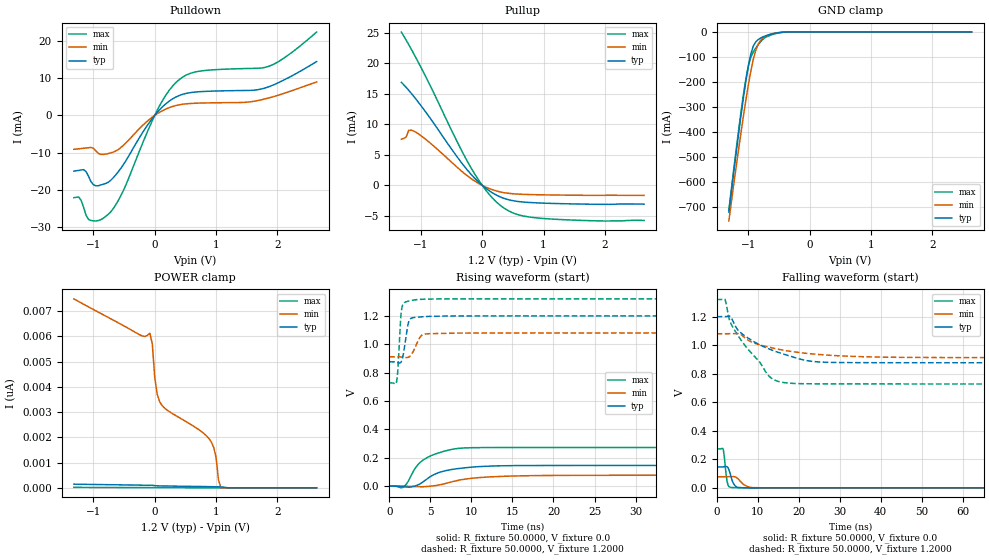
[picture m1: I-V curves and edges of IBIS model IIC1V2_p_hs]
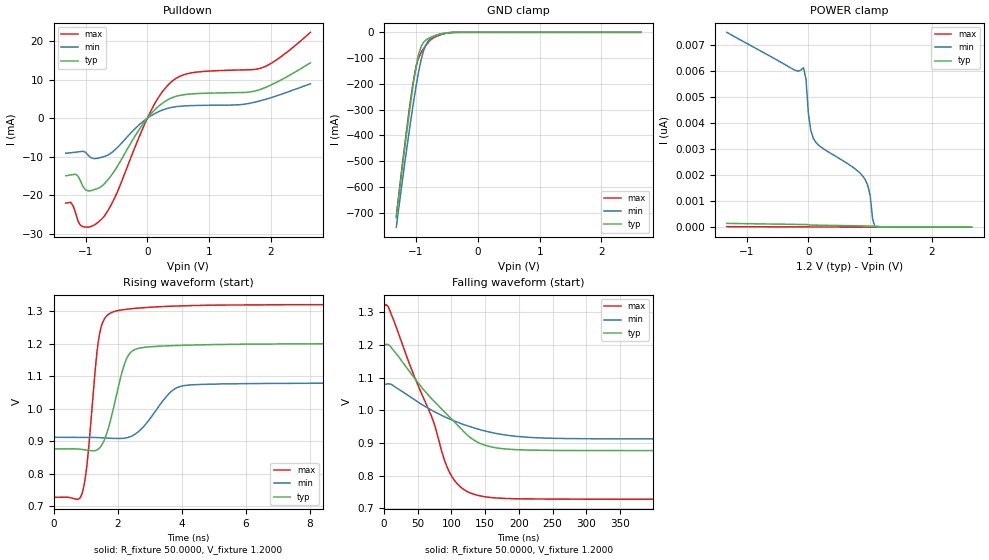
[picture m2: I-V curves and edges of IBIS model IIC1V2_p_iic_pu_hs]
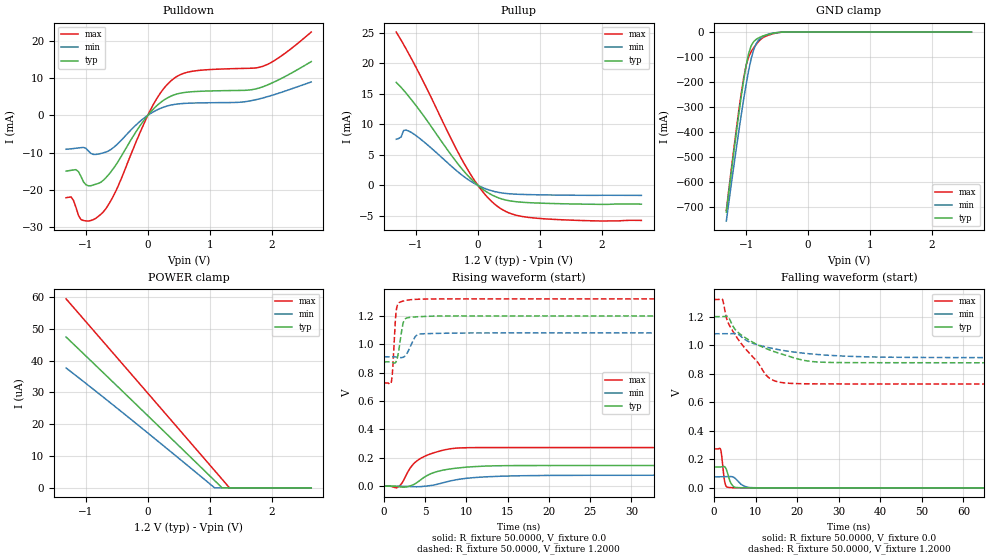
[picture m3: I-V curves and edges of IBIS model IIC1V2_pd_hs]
| IBIS file qfp64afe_1p2v.ibs generated by Viper version: 2020.12.17
[IBIS Ver]   5.0
[Comment Char]   |_char
[File Name]   qfp64afe_1p2v.ibs
[File Rev]   1.3
[Date]   Thu Dec 17 17:47:12 2020
[Source]   NXP Viper 2020.12.17
[Notes]
[Disclaimer] IMPORTANT NOTICE
  This information is provided on an AS IS basis and without warranty.
  IN NO EVENT SHALL NXP BE LIABLE FOR INCIDENTAL OR CONSEQUENTIAL
  DAMAGES ARISING FROM USE OF THIS INFORMATION. THIS DISCLAIMER OF
  WARRANTY EXTENDS TO THE USER OF THE INFORMATION, AND TO THEIR CUSTOMERS
  OR USERS OF PRODUCTS  AND IS IN LIEU OF ALL WARRANTIES WHETHER EXPRESS,
  IMPLIED, OR STATUTORY, INCLUDING IMPLIED WARRANTIES OF MERCHANTABILITY
  OR FITNESS FOR PARTICULAR PURPOSE.
  NXP does not represent or warrant that the information furnished
  hereunder is free of infringement of any third party patents,
  copyrights, trade secrets, or other intellectual property rights.
  NXP does not represent or warrant that the information is free of
  defect, or that it meets any particular standard, requirements or need
  of the user of the infomation or their customers.
  NXP reserves the right to change the information in this file
  without notice.
   http://www.nxp.com
[Copyright]   (C) Copyright NXP 2004 - 2020, All Rights Reserved.
|   qfp64Afe
[Component]   qfp64Afe
[Manufacturer]   NXP
[Package]
| variable   typ   min   max
R_pkg   0.18002   0.098036   0.22836
L_pkg   3.270e-09   2.478e-09   3.882e-09
C_pkg   4.877e-13   4.194e-13   6.388e-13
[Pin] signal_name   model_name   R_pin   L_pin   C_pin
1   P2_1   gpio   0.20176   3.768e-09 4.934e-13
2   OPAMP2_INN   NC   0.18655   3.432e-09 5.614e-13
3   P0_1   gpio   0.1882   3.425e-09 5.543e-13
4   P1_0   gpio   0.18167   3.391e-09 4.852e-13
5   ADC1IN1B   NC   0.17508   3.272e-09 4.734e-13
6   ADC1IN1A   NC   0.17211   3.184e-09 4.709e-13
7   P0_11   gpio   0.17322   3.095e-09 4.516e-13
8   VDDA   POWER   NA   NA   NA
9   VREF_OUT   NC   0.098933  2.478e-09 5.107e-13
10   VREFP   NC   0.098036  2.682e-09 4.989e-13
11   VREFN   NC   0.10339   2.593e-09 5.200e-13
12   VSSA   GND   NA   NA   NA
13   P0_16   gpio   0.18219   3.272e-09 4.683e-13
14   P0_10   gpio   0.18473   3.372e-09 4.943e-13
15   P0_15   gpio   0.1948   3.518e-09 5.647e-13
16   P0_31   gpio   0.21166   3.882e-09 5.047e-13
17   P0_8   gpio   0.19981   3.690e-09 4.818e-13
18   OPAMP0_INN   NC   0.18485   3.354e-09 5.404e-13
19   P0_27   gpio   0.1771   3.251e-09 5.158e-13
20   OPAMP1_INN   NC   0.17264   3.242e-09 4.518e-13
21   XTAL32M_N   NC   0.17308   3.207e-09 4.514e-13
22   XTAL32M_P   NC   0.17099   3.143e-09 4.435e-13
23   RESETN   gpio   0.17312   3.058e-09 4.290e-13
24   VDD_CORE   POWER   NA   NA   NA
25   P1_22   gpio   0.17347   2.976e-09 4.359e-13
26   P0_17   gpio   0.17222   3.063e-09 4.368e-13
27   P0_7   gpio   0.17974   2.960e-09 4.541e-13
28   VDDE_2   POWER   NA   NA   NA
29   VSS_MAIN_PWR   GND   NA   NA   NA
30   VSS_MAIN   GND   NA   NA   NA
31   LX   NC   0.12471   2.527e-09 6.388e-13
32   VDD_MAIN_PWR   NC   NA   NA   NA
33   XTAL32K_P   NC   0.20305   3.722e-09 4.831e-13
34   XTAL32K_N   NC   0.18797   3.388e-09 5.425e-13
35   VBAT   NC   0.17937   3.272e-09 4.763e-13
36   P0_0   gpio   0.17575   3.216e-09 4.542e-13
37   P0_9   gpio   0.17142   3.151e-09 4.522e-13
38   P0_18   gpio   0.17027   3.108e-09 4.408e-13
39   P1_13   gpio   0.17092   3.083e-09 4.194e-13
40   P1_1   gpio   0.17351   3.079e-09 4.367e-13
41   P0_26   gpio   0.17937   3.140e-09 4.480e-13
42   P1_2   gpio   0.18924   3.260e-09 4.417e-13
43   P1_3   gpio   0.20575   3.278e-09 4.623e-13
44   VDDE_4   POWER   NA   NA   NA
45   P0_24   gpio   0.18768   3.277e-09 4.591e-13
46   P0_13   iic   0.19613   3.445e-09 5.506e-13
47   P0_14   iic   0.20782   3.616e-09 5.657e-13
48   P0_20   gpio   0.21594   3.876e-09 4.850e-13
49   P0_21   gpio   0.20723   3.837e-09 4.904e-13
50   P0_22   gpio   0.1962   3.547e-09 5.661e-13
51   P0_25   gpio   0.18792   3.420e-09 5.062e-13
52   P0_2   gpio   0.18663   3.397e-09 4.750e-13
53   P1_15   gpio   0.17882   3.273e-09 4.700e-13
54   P0_19   gpio   0.17446   3.156e-09 4.633e-13
55   P0_3   gpio   0.17673   3.008e-09 4.457e-13
56   VDDE_4   POWER   NA   NA   NA
57   P0_4   gpio   0.17637   3.003e-09 4.457e-13
58   P1_16   gpio   0.17537   3.170e-09 4.476e-13
59   P0_6   gpio   0.17935   3.248e-09 4.687e-13
60   P0_5   gpio   0.18758   3.378e-09 4.757e-13
61   P0_29   gpio   0.19171   3.430e-09 4.834e-13
62   P1_11   gpio   0.20582   3.539e-09 5.647e-13
63   P0_30   gpio   0.22836   3.428e-09 5.818e-13
64   VDDE_4   POWER   NA   NA   NA
65   VSS   GND   NA   NA   NA
[Pin Mapping]   pulldown_ref   pullup_ref
1   VSS   VDDA
2   NC   NC
3   VSS   VDDA
4   VSS   VDDA
5   NC   NC
6   NC   NC
7   VSS   VDDA
8   NC   VDDA
9   NC   NC
10   NC   NC
11   NC   NC
12   VSSA   NC
13   VSS   VDDA
14   VSS   VDDA
15   VSS   VDDA
16   VSS   VDDA
17   VSS   VDDA
18   NC   NC
19   VSS   VDDA
20   NC   NC
21   NC   NC
22   NC   NC
23   VSS   VDDE_2
24   NC   VDD_CORE
25   VSS   VDDE_2
26   VSS   VDDE_2
27   VSS   VDDE_2
28   NC   VDDE_2
29   VSS_MAIN_PWR   NC
30   VSS_MAIN   NC
31   NC   NC
32   NC   NC
33   NC   NC
34   NC   NC
35   NC   NC
36   VSS   VDDE_4
37   VSS   VDDE_4
38   VSS   VDDE_4
39   VSS   VDDE_4
40   VSS   VDDE_4
41   VSS   VDDE_4
42   VSS   VDDE_4
43   VSS   VDDE_4
44   NC   VDDE_4
45   VSS   VDDE_4
46   VSS   VDDE_4
47   VSS   VDDE_4
48   VSS   VDDE_4
49   VSS   VDDE_4
50   VSS   VDDE_4
51   VSS   VDDE_4
52   VSS   VDDE_4
53   VSS   VDDE_4
54   VSS   VDDE_4
55   VSS   VDDE_4
56   NC   VDDE_4
57   VSS   VDDE_4
58   VSS   VDDE_4
59   VSS   VDDE_4
60   VSS   VDDE_4
61   VSS   VDDE_4
62   VSS   VDDE_4
63   VSS   VDDE_4
64   NC   VDDE_4
65   VSS   NC
|*   Model Selector   *
[Model Selector] gpio
MFIO1V2_pd_hs   EPUN=1 EPD=1 EHS=1
MFIO1V2_pd_ls   EPUN=1 EPD=1 EHS=0
MFIO1V2_pu_hs   EPUN=0 EPD=0 EHS=1
MFIO1V2_pu_ls   EPUN=0 EPD=0 EHS=0
MFIO1V2_p_hs   EPUN=1 EPD=0 EHS=1
MFIO1V2_p_ls   EPUN=1 EPD=0 EHS=0
MFIO1V2_r_hs   EPUN=0 EPD=1 EHS=1
MFIO1V2_r_ls   EPUN=0 EPD=1 EHS=0
[Model Selector] iic
IIC1V2_pd_hs   EGP=1 EPUN=1 EPD=1 EHS=1
IIC1V2_pd_ls   EGP=1 EPUN=1 EPD=1 EHS=0
IIC1V2_p_hs   EGP=1 EPUN=1 EPD=0 EHS=1
IIC1V2_p_ls   EGP=1 EPUN=1 EPD=0 EHS=0
IIC1V2_pu_hs   EGP=1 EPUN=0 EPD=0 EHS=1
IIC1V2_pu_ls   EGP=1 EPUN=0 EPD=0 EHS=0
IIC1V2_r_hs   EGP=1 EPUN=0 EPD=1 EHS=1
IIC1V2_r_ls   EGP=1 EPUN=0 EPD=1 EHS=0
IIC1V2_pd_iic_hs   EGP=0 ECS=0 EPUN=1 EPD=1
IIC1V2_p_iic_hs   EGP=0 ECS=0 EPUN=1 EPD=0
IIC1V2_pu_iic_hs   EGP=0 ECS=0 EPUN=0 EPD=0
IIC1V2_r_iic_hs   EGP=0 ECS=0 EPUN=0 EPD=1
IIC1V2_pd_iic_pu_hs   EGP=0 ECS=1 EPUN=1 EPD=1 SSEL=1
IIC1V2_p_iic_pu_hs   EGP=0 ECS=1 EPUN=1 EPD=0 SSEL=1
IIC1V2_pu_iic_pu_hs   EGP=0 ECS=1 EPUN=0 EPD=0 SSEL=1
IIC1V2_r_iic_pu_hs   EGP=0 ECS=1 EPUN=0 EPD=1 SSEL=1
| End [Component] qfp64Afe
| Models and submodels in the file (24): IIC1V2_p_hs (I/O), IIC1V2_p_iic_hs (I/O_open_drain), IIC1V2_p_iic_pu_hs (I/O_open_drain), IIC1V2_p_ls (I/O), IIC1V2_pd_hs (I/O), IIC1V2_pd_iic_hs (I/O_open_drain), IIC1V2_pd_iic_pu_hs (I/O_open_drain), IIC1V2_pd_ls (I/O), IIC1V2_pu_hs (I/O), IIC1V2_pu_iic_hs (I/O_open_drain), IIC1V2_pu_iic_pu_hs (I/O_open_drain), IIC1V2_pu_ls (I/O), IIC1V2_r_hs (I/O), IIC1V2_r_iic_hs (I/O_open_drain), IIC1V2_r_iic_pu_hs (I/O_open_drain), IIC1V2_r_ls (I/O), MFIO1V2_p_hs (I/O), MFIO1V2_p_ls (I/O), MFIO1V2_pd_hs (I/O), MFIO1V2_pd_ls (I/O), MFIO1V2_pu_hs (I/O), MFIO1V2_pu_ls (I/O), MFIO1V2_r_hs (I/O), MFIO1V2_r_ls (I/O)
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[Model] IIC1V2_p_hs
|   Model IIC1V2_p_hs
| This model was characterised for following simulation conditions:
| External (pad) voltage:
|   - Typ: 1.2V,   - Min: 1.08V,   - Max: 1.32V
| Library cells for typ/min/max conditions are connected as defined below:
|  IO - External Pad
|  A - Core Input
|  EN - Output Buffer Enable
|  BOOST - vdde
|  EGP - vdd
|  EHS - vdd
|  ENZI - vdd
|  EPD - gnd
|  EPUN - vdd
|  ZI - NC
|  ZIF - NC
|  gnd - gnd
|  gnde - gnde
|  vdd - vdd
|  vdde - vdde
| All other pins connected to ground
Model_type I/O
Polarity   Non-Inverting
Enable   Active-Low
Vinl =   0.5400V
Vinh =   1.2600V
Vmeas =  0.9000V
Cref =   0.0F
Rref =   1.0000k
Vref =   0.0V
C_comp   3.6473pF   3.5138pF   3.7665pF
|C_comp_pullup   0.9539pF   0.9082pF   0.9728pF
|C_comp_pulldown   2.3399pF   2.4915pF   2.1962pF
[Model Spec]
| variable   typ   min   max
Vinh   0.3600V   0.3240V   0.3960V
Vinl   0.8400V   0.7560V   0.9240V
Vmeas   0.6000V   0.5400V   0.6600V
[Temperature Range]   25.0000   0.1250k   -40.0000
[Voltage Range]   1.2000V   1.0800V   1.3200V
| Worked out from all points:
|   slope of the pulldown table from 0 to 0.18 V, typ, clamps not added: 58.3 ohm
|   slope of the pullup table from 0 to 0.18 V, typ, clamps not added: 138 ohm
|   GND clamp passes 1 mA (typ) near -0.45 V on its own axis
|   rising waveform, R_fixture 50.0000, V_fixture 0.0: 20-80 % time 3.45ns typ, 4.61ns min, 2.73ns max; typ from 0 V to 0.146 V
|   rising waveform, R_fixture 50.0000, V_fixture 1.2000: 20-80 % time 519ps typ, 830ps min, 343ps max; typ from 0.877 V to 1.2 V
|   falling waveform, R_fixture 50.0000, V_fixture 0.0: 20-80 % time 1.02ns typ, 1.79ns min, 624ps max; typ from 0.146 V to 0 V
|   falling waveform, R_fixture 50.0000, V_fixture 1.2000: 20-80 % time 11.4ns typ, 13.9ns min, 8.37ns max; typ from 1.2 V to 0.877 V
[Pulldown]
|Voltage   I(typ)   I(min)   I(max)
-1.32V    -14.96mA   -9.099mA   -22.09mA
-1.24V    -14.75mA   -8.982mA   -21.89mA
-1.16V    -14.56mA   -8.83mA    -24.7mA
-1.04V    -17.82mA   -8.609mA   -28.21mA
-920mV    -18.88mA   -10.21mA   -28.21mA
-720mV    -17.44mA   -10.07mA   -25.94mA
-520mV    -13.41mA   -8.157mA   -20.44mA
80mV      1.521mA    840uA      2.628mA
440mV     5.569mA    2.951mA    10.1mA
760mV     6.377mA    3.307mA    11.92mA
1.84V     7.559mA    4.586mA    13.06mA
2.64V     14.43mA    8.958mA    22.36mA
[Pullup]
|Voltage   I(typ)   I(min)   I(max)
-1.32V    16.87mA    7.562mA    25.11mA
-1.24V    16.04mA    7.944mA    23.76mA
-1.2V     15.58mA    9.001mA    23.05mA
-1.08V    14.1mA     8.693mA    20.85mA
-400mV    4.54mA     2.884mA    6.955mA
-200mV    2.009mA    1.241mA    3.176mA
80mV      -640.3uA   -373.7uA   -1.07mA
320mV     -1.996mA   -1.123mA   -3.467mA
560mV     -2.602mA   -1.412mA   -4.719mA
920mV     -2.876mA   -1.532mA   -5.352mA
1.96V     -3.103mA   -1.628mA   -5.823mA
2.64V     -3.069mA   -1.636mA   -5.736mA
[GND_clamp]
|Voltage   I(typ)   I(min)   I(max)
-1.32V    -720.7mA   -756.4mA   -713.8mA
-1.12V    -330.9mA   -399.5mA   -316.8mA
-1.04V    -192.4mA   -269.2mA   -184.4mA
-1V       -133.6mA   -209.3mA   -133.5mA
-960mV    -86.73mA   -154.7mA   -99.45mA
-920mV    -55.68mA   -108.2mA   -79.01mA
-880mV    -39.01mA   -72.34mA   -63.7mA
-840mV    -29.9mA    -47.99mA   -50.25mA
-760mV    -18.92mA   -23.38mA   -28.31mA
-640mV    -9.212mA   -8.622mA   -12.72mA
-400mV    -328.4uA   -396.6uA   -434.3uA
2.64V     0A         0A         0A
[POWER_clamp]
|Voltage   I(typ)   I(min)   I(max)
-1.32V    146.2pA    7.487nA    20.6pA
-240mV    107.2pA    6.058nA    10.71pA
-80mV     104.3pA    6.128nA    10.43pA
-40mV     105.3pA    5.7nA      9.002pA
0V        87.49pA    4.363nA    8.131pA
80mV      77.4pA     3.412nA    7.54pA
880mV     48.09pA    1.964nA    2.626pA
960mV     44.51pA    1.611nA    2.139pA
1V        42.37pA    1.211nA    1.894pA
1.04V     39.75pA    304.3pA    1.646pA
1.08V     36.09pA    0A         1.394pA
2.64V     0A         0A         0A
[Ramp]
| variable   typ   min   max
dV/dt_r  87.7543m/3.4464n   46.4153m/4.6065n   0.1637/2.7335n
dV/dt_f  0.1940/11.3751n   0.1007/13.8710n   0.3553/8.3673n
R_load = 50.0000
[Rising Waveform]
R_fixture= 50.0000
V_fixture= 0.0
V_fixture_min= 0.0
V_fixture_max= 0.0
|time   V(typ)   V(min)   V(max)
0s        663.7pV    60.46nV    39.17pV
1.735ns   -2.682mV   172.8uV    -4.698mV
2.17ns    -6.221mV   31.22uV    20.88mV
3.005ns   -724.5uV   -2.28mV    111.7mV
3.546ns   10.08mV    -3.777mV   154.7mV
5.333ns   78.4mV     2.145mV    220.8mV
8.076ns   122mV      37.42mV    264mV
11.88ns   140.8mV    64.41mV    272.4mV
33.26ns   146.2mV    77.18mV    272.7mV
1us       146.3mV    77.36mV    272.8mV
[Rising Waveform]
R_fixture= 50.0000
V_fixture= 1.2000
V_fixture_min= 1.0800
V_fixture_max= 1.3200
|time   V(typ)   V(min)   V(max)
0s        876.6mV    912.2mV    727.9mV
925.4ps   873.7mV    912.5mV    744.3mV
1.07ns    870.9mV    912.4mV    833.7mV
1.417ns   872.4mV    910.7mV    1.195V
1.686ns   919.9mV    908.8mV    1.282V
2.223ns   1.121V     906.8mV    1.303V
2.507ns   1.175V     914.8mV    1.307V
3.963ns   1.194V     1.064V     1.317V
5.617ns   1.198V     1.076V     1.319V
1us       1.2V       1.08V      1.32V
[Falling Waveform]
R_fixture= 50.0000
V_fixture= 0.0
V_fixture_min= 0.0
V_fixture_max= 0.0
|time   V(typ)   V(min)   V(max)
0s        146.3mV    77.36mV    272.8mV
1.583ns   146.6mV    77.35mV    269.1mV
1.815ns   147.6mV    77.32mV    228.9mV
2.378ns   149.7mV    77.32mV    73.57mV
2.869ns   135mV      77.95mV    12.66mV
4.132ns   28.89mV    79.27mV    1.543mV
5.749ns   1.763mV    46.03mV    353.1uV
8.143ns   287.7uV    3.769mV    70.4uV
13.48ns   24.82uV    120.4uV    7.14uV
1us       23.59nV    99.24nV    13.67nV
[Falling Waveform]
R_fixture= 50.0000
V_fixture= 1.2000
V_fixture_min= 1.0800
V_fixture_max= 1.3200
|time   V(typ)   V(min)   V(max)
0s        1.2V       1.08V      1.32V
1.968ns   1.2V       1.08V      1.323V
3.029ns   1.203V     1.08V      1.186V
3.948ns   1.169V     1.08V      1.125V
6.283ns   1.078V     1.066V     1.021V
12.91ns   971.7mV    984.4mV    779.2mV
15.66ns   943.4mV    967.9mV    741.4mV
21.16ns   896.8mV    945.1mV    729.9mV
62.12ns   876.8mV    912.9mV    728mV
1us       876.6mV    912.2mV    727.9mV
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[Model] IIC1V2_p_iic_pu_hs
|   Model IIC1V2_p_iic_pu_hs
| This model was characterised for following simulation conditions:
| External (pad) voltage:
|   - Typ: 1.2V,   - Min: 1.08V,   - Max: 1.32V
| Library cells for typ/min/max conditions are connected as defined below:
|  IO - External Pad
|  A - Core Input
|  EN - Output Buffer Enable
|  BOOST - vdde
|  ECS - vdd
|  EGP - gnd
|  ENZI - vdd
|  EPD - gnd
|  EPUN - vdd
|  SSEL - vdd
|  ZI - NC
|  ZIF - NC
|  gnd - gnd
|  gnde - gnde
|  vdd - vdd
|  vdde - vdde
| All other pins connected to ground
Model_type I/O_open_drain
Polarity   Non-Inverting
Enable   Active-Low
Vinl =   0.5400V
Vinh =   1.2600V
Vmeas =  0.9000V
Cref =   0.0F
Rref =   1.0000k
Vref =   1.2000V
C_comp   3.6473pF   3.5138pF   3.7665pF
|C_comp_pullup   0.9537pF   0.9078pF   0.9727pF
|C_comp_pulldown   2.3401pF   2.4920pF   2.1963pF
[Model Spec]
| variable   typ   min   max
Vinh   0.3600V   0.3240V   0.3960V
Vinl   0.8400V   0.7560V   0.9240V
Vmeas   0.6000V   0.5400V   0.6600V
Vref   1.2000V   1.0800V   1.3200V
Cref   0.0F   0.0F   0.0F
Rref   1.0000k   1.0000k   1.0000k
[Temperature Range]   25.0000   0.1250k   -40.0000
[Voltage Range]   1.2000V   1.0800V   1.3200V
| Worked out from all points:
|   slope of the pulldown table from 0 to 0.18 V, typ, clamps not added: 58.3 ohm
|   GND clamp passes 1 mA (typ) near -0.45 V on its own axis
|   rising waveform, R_fixture 50.0000, V_fixture 1.2000: 20-80 % time 494ps typ, 787ps min, 328ps max; typ from 0.877 V to 1.2 V
|   falling waveform, R_fixture 50.0000, V_fixture 1.2000: 20-80 % time 83.3ns typ, 99ns min, 62.7ns max; typ from 1.2 V to 0.877 V
[Pulldown]
|Voltage   I(typ)   I(min)   I(max)
-1.32V    -14.96mA   -9.099mA   -22.09mA
-1.24V    -14.75mA   -8.982mA   -21.89mA
-1.16V    -14.56mA   -8.83mA    -24.7mA
-1.04V    -17.82mA   -8.609mA   -28.21mA
-920mV    -18.88mA   -10.21mA   -28.21mA
-720mV    -17.44mA   -10.07mA   -25.94mA
-520mV    -13.41mA   -8.157mA   -20.44mA
80mV      1.521mA    840uA      2.628mA
440mV     5.569mA    2.951mA    10.1mA
760mV     6.377mA    3.307mA    11.92mA
1.84V     7.559mA    4.586mA    13.06mA
2.64V     14.43mA    8.958mA    22.36mA
[GND_clamp]
|Voltage   I(typ)   I(min)   I(max)
-1.32V    -720.7mA   -756.4mA   -713.8mA
-1.12V    -330.9mA   -399.5mA   -316.8mA
-1.04V    -192.4mA   -269.2mA   -184.4mA
-1V       -133.6mA   -209.3mA   -133.5mA
-960mV    -86.73mA   -154.7mA   -99.45mA
-920mV    -55.68mA   -108.2mA   -79.01mA
-880mV    -39.01mA   -72.34mA   -63.7mA
-840mV    -29.9mA    -47.99mA   -50.25mA
-760mV    -18.92mA   -23.38mA   -28.31mA
-640mV    -9.212mA   -8.622mA   -12.72mA
-400mV    -328.4uA   -396.6uA   -434.3uA
2.64V     0A         0A         0A
[POWER_clamp]
|Voltage   I(typ)   I(min)   I(max)
-1.32V    146.2pA    7.487nA    20.6pA
-240mV    107.2pA    6.058nA    10.71pA
-80mV     104.3pA    6.128nA    10.43pA
-40mV     105.3pA    5.7nA      9.002pA
0V        87.49pA    4.363nA    8.131pA
80mV      77.4pA     3.412nA    7.54pA
880mV     48.09pA    1.964nA    2.626pA
960mV     44.51pA    1.611nA    2.139pA
1V        42.37pA    1.211nA    1.894pA
1.04V     39.75pA    304.3pA    1.646pA
1.08V     36.09pA    0A         1.394pA
2.64V     0A         0A         0A
[Ramp]
| variable   typ   min   max
dV/dt_r  0.1940/0.4944n   0.1007/0.7878n   0.3553/0.3284n
dV/dt_f  0.1940/83.2985n   0.1006/99.0257n   0.3552/62.6594n
R_load = 50.0000
[Rising Waveform]
R_fixture= 50.0000
V_fixture= 1.2000
V_fixture_min= 1.0800
V_fixture_max= 1.3200
|time   V(typ)   V(min)   V(max)
0s        876.6mV    912.2mV    727.9mV
903ps     874.8mV    912.4mV    743.6mV
1.063ns   872.6mV    912.3mV    844.4mV
1.396ns   875.6mV    911.2mV    1.204V
1.672ns   926.9mV    909.9mV    1.286V
2.162ns   1.12V      908.9mV    1.304V
2.467ns   1.178V     917.2mV    1.308V
3.862ns   1.194V     1.065V     1.315V
6.142ns   1.198V     1.077V     1.319V
1us       1.2V       1.08V      1.32V
[Falling Waveform]
R_fixture= 50.0000
V_fixture= 1.2000
V_fixture_min= 1.0800
V_fixture_max= 1.3200
|time   V(typ)   V(min)   V(max)
0s        1.2V       1.08V      1.32V
6.561ns   1.2V       1.081V     1.316V
45.2ns    1.098V     1.032V     1.102V
69.62ns   1.038V     1.002V     985.8mV
95.52ns   983.6mV    975.1mV    817.3mV
112.5ns   947.2mV    961mV      767.4mV
135.3ns   906.9mV    945.2mV    742.1mV
177.8ns   882.4mV    925.3mV    730.9mV
264.1ns   877.4mV    914.1mV    728.5mV
1us       876.7mV    912.3mV    728mV
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[Model] IIC1V2_pd_hs
|   Model IIC1V2_pd_hs
| This model was characterised for following simulation conditions:
| External (pad) voltage:
|   - Typ: 1.2V,   - Min: 1.08V,   - Max: 1.32V
| Library cells for typ/min/max conditions are connected as defined below:
|  IO - External Pad
|  A - Core Input
|  EN - Output Buffer Enable
|  BOOST - vdde
|  EGP - vdd
|  EHS - vdd
|  ENZI - vdd
|  EPD - vdd
|  EPUN - vdd
|  ZI - NC
|  ZIF - NC
|  gnd - gnd
|  gnde - gnde
|  vdd - vdd
|  vdde - vdde
| All other pins connected to ground
Model_type I/O
Polarity   Non-Inverting
Enable   Active-Low
Vinl =   0.5400V
Vinh =   1.2600V
Vmeas =  0.9000V
Cref =   0.0F
Rref =   1.0000k
Vref =   0.0V
C_comp   3.6164pF   3.4768pF   3.7417pF
|C_comp_pullup   0.9404pF   0.8996pF   0.9549pF
|C_comp_pulldown   2.3238pF   2.4767pF   2.1786pF
[Model Spec]
| variable   typ   min   max
Vinh   0.3600V   0.3240V   0.3960V
Vinl   0.8400V   0.7560V   0.9240V
Vmeas   0.6000V   0.5400V   0.6600V
[Temperature Range]   25.0000   0.1250k   -40.0000
[Voltage Range]   1.2000V   1.0800V   1.3200V
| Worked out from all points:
|   slope of the pulldown table from 0 to 0.18 V, typ, clamps not added: 58.3 ohm
|   slope of the pullup table from 0 to 0.18 V, typ, clamps not added: 138 ohm
|   GND clamp passes 1 mA (typ) near -0.45 V on its own axis
|   rising waveform, R_fixture 50.0000, V_fixture 0.0: 20-80 % time 3.43ns typ, 4.6ns min, 2.73ns max; typ from 0 V to 0.146 V
|   rising waveform, R_fixture 50.0000, V_fixture 1.2000: 20-80 % time 519ps typ, 831ps min, 343ps max; typ from 0.876 V to 1.2 V
|   falling waveform, R_fixture 50.0000, V_fixture 0.0: 20-80 % time 1.02ns typ, 1.79ns min, 624ps max; typ from 0.146 V to 0 V
|   falling waveform, R_fixture 50.0000, V_fixture 1.2000: 20-80 % time 11.4ns typ, 13.8ns min, 8.35ns max; typ from 1.2 V to 0.876 V
[Pulldown]
|Voltage   I(typ)   I(min)   I(max)
-1.32V    -14.96mA   -9.099mA   -22.09mA
-1.24V    -14.75mA   -8.982mA   -21.89mA
-1.16V    -14.56mA   -8.83mA    -24.7mA
-1.04V    -17.82mA   -8.609mA   -28.21mA
-920mV    -18.88mA   -10.21mA   -28.21mA
-720mV    -17.44mA   -10.07mA   -25.94mA
-520mV    -13.41mA   -8.157mA   -20.44mA
80mV      1.521mA    840uA      2.628mA
440mV     5.569mA    2.951mA    10.1mA
760mV     6.377mA    3.307mA    11.92mA
1.84V     7.555mA    4.581mA    13.06mA
2.64V     14.41mA    8.944mA    22.34mA
[Pullup]
|Voltage   I(typ)   I(min)   I(max)
-1.32V    16.86mA    7.551mA    25.1mA
-1.24V    16.02mA    7.934mA    23.74mA
-1.2V     15.57mA    8.991mA    23.04mA
-1.08V    14.09mA    8.684mA    20.84mA
-400mV    4.539mA    2.883mA    6.954mA
-200mV    2.009mA    1.241mA    3.176mA
80mV      -640.3uA   -373.7uA   -1.07mA
320mV     -1.996mA   -1.123mA   -3.467mA
560mV     -2.602mA   -1.412mA   -4.719mA
920mV     -2.876mA   -1.532mA   -5.352mA
1.96V     -3.103mA   -1.628mA   -5.823mA
2.64V     -3.069mA   -1.636mA   -5.736mA
[GND_clamp]
|Voltage   I(typ)   I(min)   I(max)
-1.32V    -720.7mA   -756.5mA   -713.8mA
-1.12V    -330.9mA   -399.5mA   -316.8mA
-1.04V    -192.4mA   -269.2mA   -184.4mA
-1V       -133.6mA   -209.3mA   -133.5mA
-960mV    -86.74mA   -154.7mA   -99.46mA
-920mV    -55.69mA   -108.2mA   -79.02mA
-880mV    -39.02mA   -72.35mA   -63.71mA
-840mV    -29.9mA    -48mA      -50.26mA
-760mV    -18.93mA   -23.39mA   -28.32mA
-640mV    -9.22mA    -8.628mA   -12.73mA
-400mV    -335.3uA   -402.3uA   -442.6uA
2.64V     0A         0A         0A
[POWER_clamp]
|Voltage   I(typ)   I(min)   I(max)
-1.32V    47.4uA     37.67uA    59.39uA
-280mV    27.94uA    21.65uA    36.04uA
1.08V     2.274uA    0A         5.413uA
1.2V      0A         0A         2.707uA
1.32V     0A         0A         0A
2.64V     0A         0A         0A
[Ramp]
| variable   typ   min   max
dV/dt_r  87.6725m/3.4349n   46.3783m/4.5961n   0.1635/2.7265n
dV/dt_f  0.1940/11.3621n   0.1007/13.8533n   0.3552/8.3552n
R_load = 50.0000
[Rising Waveform]
R_fixture= 50.0000
V_fixture= 0.0
V_fixture_min= 0.0
V_fixture_max= 0.0
|time   V(typ)   V(min)   V(max)
0s        642.2pV    57.99nV    36.63pV
1.694ns   -2.271mV   170.4uV    -6.391mV
2.176ns   -6.251mV   22.34uV    21.45mV
3.018ns   -498.8uV   -2.34mV    113mV
3.566ns   10.64mV    -3.8mV     156.1mV
5.371ns   79.64mV    2.414mV    221.6mV
7.998ns   121.3mV    36.42mV    263.3mV
11.68ns   140.2mV    63.76mV    272.1mV
33.54ns   146.1mV    77.12mV    272.4mV
1us       146.1mV    77.3mV     272.5mV
[Rising Waveform]
R_fixture= 50.0000
V_fixture= 1.2000
V_fixture_min= 1.0800
V_fixture_max= 1.3200
|time   V(typ)   V(min)   V(max)
0s        875.8mV    911.4mV    727.2mV
906.2ps   873.2mV    911.8mV    737.4mV
1.073ns   870mV      911.7mV    835.3mV
1.421ns   871.9mV    909.9mV    1.198V
1.691ns   920.7mV    908mV      1.282V
2.233ns   1.123V     906.2mV    1.302V
2.514ns   1.175V     914.6mV    1.306V
3.919ns   1.193V     1.061V     1.316V
5.546ns   1.197V     1.075V     1.318V
1us       1.199V     1.079V     1.319V
[Falling Waveform]
R_fixture= 50.0000
V_fixture= 0.0
V_fixture_min= 0.0
V_fixture_max= 0.0
|time   V(typ)   V(min)   V(max)
0s        146.1mV    77.3mV     272.5mV
1.573ns   146.4mV    77.29mV    269.6mV
1.822ns   147.5mV    77.26mV    227mV
2.382ns   149.5mV    77.26mV    72.39mV
2.876ns   134.4mV    77.9mV     12.14mV
4.152ns   27.81mV    79.14mV    1.429mV
5.775ns   1.661mV    45.1mV     306.5uV
8.109ns   267.7uV    3.938mV    54.94uV
13.4ns    20.27uV    113.7uV    4.825uV
1us       23.56nV    96.75nV    13.66nV
[Falling Waveform]
R_fixture= 50.0000
V_fixture= 1.2000
V_fixture_min= 1.0800
V_fixture_max= 1.3200
|time   V(typ)   V(min)   V(max)
0s        1.199V     1.079V     1.319V
1.975ns   1.199V     1.079V     1.322V
3.038ns   1.202V     1.079V     1.184V
3.832ns   1.175V     1.079V     1.13V
5.997ns   1.083V     1.073V     1.032V
12.59ns   974.3mV    985.8mV    787.2mV
15.19ns   947mV      969.7mV    743.7mV
20.75ns   898.6mV    945.5mV    729.4mV
63.98ns   876mV      912.1mV    727.3mV
1us       875.8mV    911.5mV    727.2mV
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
